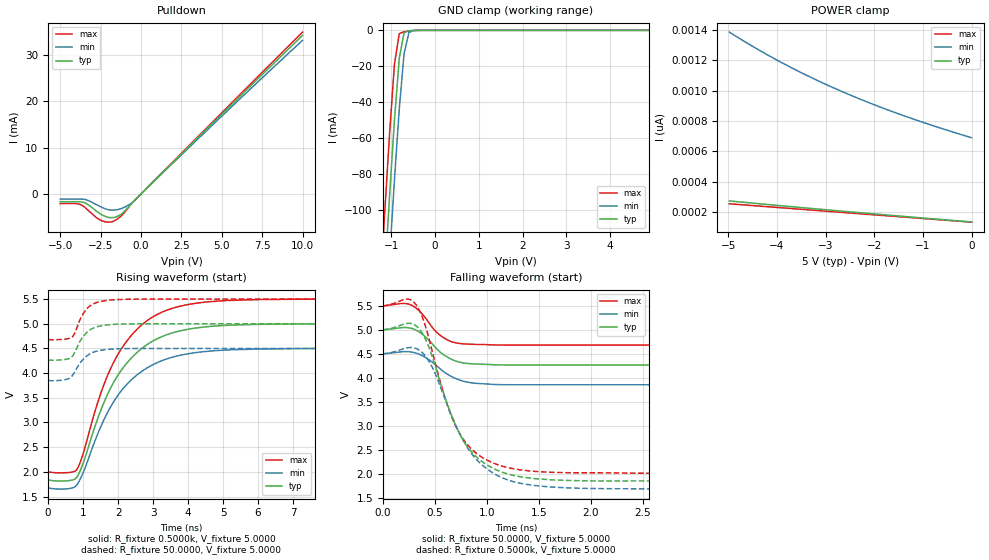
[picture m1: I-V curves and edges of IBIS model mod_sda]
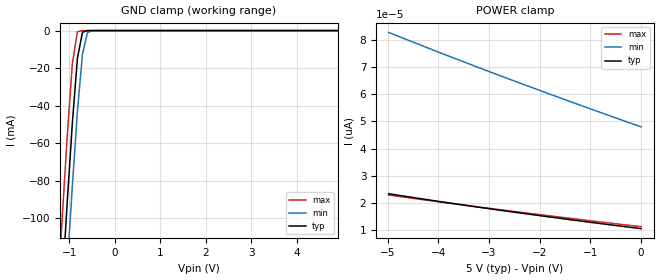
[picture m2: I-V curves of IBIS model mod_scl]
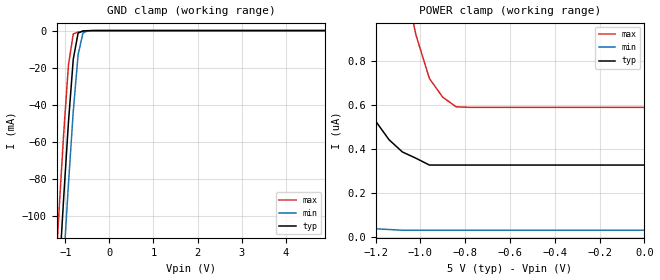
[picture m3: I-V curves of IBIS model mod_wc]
| IBIS (I/O, Buffer, Information, Specification) Model, officially
| electronic behavioral standard for Buffer structures of digital pins.
[IBIS ver]  4.0
[File name] m24c16_fc3_tssop8.ibs
[File Rev]  1.0
[Date]   24 Sept 2014
[Source]   CAD & Design Services (Catania) - STMicroelectronics
[Notes]
   (Note1)  This IBIS model includes the TSSOP8 package data
   (Note2)  This IBIS model has some Notes about the non-monotonicity
   of the I-V curves, but they are not indicative of problems
   inside the model;
[Copyright] (c) 2014 STMicroelectronics
|   Component M24C16
[Component] M24C16
[Manufacturer] STMicroelectronics
[Package]
| variable   typ   min   max
R_pkg   0.0   0.0   0.0
L_pkg   0.0H   0.0H   0.0H
C_pkg   0.0F   0.0F   0.0F
[Pin]  signal_name   model_name   R_pin   L_pin   C_pin
1   1NC   NC   NA   NA   NA
2   2NC   NC   NA   NA   NA
3   3NC   NC   NA   NA   NA
4   VSS   GND   NA   NA   NA
5   SDA   mod_sda   NA   NA   NA
6   SCL   mod_scl   NA   NA   NA
7   WCN   mod_wc   NA   NA   NA
8   VCC   POWER   NA   NA   NA
[Package Model]  182696_TSSOP8
[Define Package Model]  182696_TSSOP8
[Manufacturer]  STMicroelectronics
[OEM]  STMicroelectronics
[Description]  8 pin TSSOP package
[Number Of Pins]  8
[Pin Numbers]
|Pin Num   Terminal Name
1   | net1
2   | net2
3   | net3
4   | net4_GND
5   | net5
6   | net6
7   | net7
8   | net8_VDD
[Model Data]
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[End Model Data]
[End Package Model]
| Models and submodels in the file (3): mod_sda (I/O_open_drain), mod_scl (Input), mod_wc (Input)
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|   Model mod_sda
[Model]   mod_sda
Model_type I/O_open_drain
Polarity   Inverting
Vinl   =   1.500V
Vinh   =   3.500V
Vmeas  =   2.500V
Cref   =   10pF
Rref   =   1k
Vref   =   5.000V
C_comp   1.845pF   1.683pF   1.932pF
[Temperature Range]  25.0000   85.0000   -40.0000
[Voltage Range]   5.0000V   4.5000V   5.5000V
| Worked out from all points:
|   slope of the pulldown table from 0 to 0.75 V, typ, clamps not added: 290 ohm
|   GND clamp passes 1 mA (typ) near -0.68 V on its own axis
|   rising waveform, R_fixture 0.5000k, V_fixture 5.0000: 20-80 % time 1.33ns typ, 1.36ns min, 1.29ns max; typ from 1.83 V to 5 V
|   rising waveform, R_fixture 50.0000, V_fixture 5.0000: 20-80 % time 396ps typ, 424ps min, 373ps max; typ from 4.27 V to 5 V
|   falling waveform, R_fixture 50.0000, V_fixture 5.0000: 20-80 % time 226ps typ, 256ps min, 202ps max; typ from 5 V to 4.27 V
|   falling waveform, R_fixture 0.5000k, V_fixture 5.0000: 20-80 % time 361ps typ, 392ps min, 333ps max; typ from 5 V to 1.83 V
[Pulldown]
|Voltage   I(typ)   I(min)   I(max)
-5V       -1.67mA    -1.12mA    -2.076mA
-4.04V    -1.67mA    -1.12mA    -2.076mA
-3.72V    -1.69mA    -1.124mA   -2.322mA
-3.4V     -2.033mA   -1.24mA    -3.126mA
-2.76V    -3.71mA    -2.317mA   -5.101mA
-2.28V    -4.74mA    -3.122mA   -5.95mA
-1.8V     -5.117mA   -3.496mA   -6.006mA
-1.48V    -4.87mA    -3.399mA   -5.446mA
-1.16V    -4.184mA   -3.077mA   -4.516mA
-520mV    -1.838mA   -1.762mA   -1.845mA
5.24V     18.02mA    17.57mA    18.34mA
10V       34.18mA    33.1mA     34.88mA
[GND_clamp]
|Voltage   I(typ)   I(min)   I(max)
-5V       -1.825A    -1.857A    -1.794A
-1.26V    -181mA     -216.2mA   -145.7mA
-1.15V    -135.5mA   -170.6mA   -100.2mA
-1.04V    -91.23mA   -126mA     -56.63mA
-930mV    -49.7mA    -83.07mA   -18.72mA
-820mV    -15.43mA   -43.63mA   -1.793mA
-710mV    -1.308mA   -12.96mA   -800.3uA
-600mV    -197.9uA   -1.278mA   -438.8uA
-490mV    -52.7uA    -150.8uA   -129uA
4.9V      130.6pA    728.2pA    117.6pA
[POWER_clamp]
|Voltage   I(typ)   I(min)   I(max)
-4.98V    272.3pA    1.386nA    253.4pA
-4.44V    256pA      1.28nA     240.1pA
-3.84V    238.3pA    1.174nA    225.3pA
-3.3V     222.7pA    1.087nA    212.1pA
-2.7V     205.8pA    998.7pA    197.5pA
-2.04V    187.6pA    911.4pA    181.4pA
-1.38V    169.7pA    832.6pA    165.4pA
-660mV    150.5pA    754.6pA    148pA
0V        133.2pA    689.1pA    132pA
[Ramp]
| variable   typ   min   max
dV/dt_r   0.4405/0.4439n   0.3885/0.4693n   0.4915/0.4754n
dV/dt_f   0.4405/0.2435n   0.3885/0.2716n   0.4915/0.2233n
R_load = 50.0000
[Rising Waveform]
R_fixture= 0.5000k
V_fixture= 5.0000
V_fixture_min= 4.5000
V_fixture_max= 5.5000
|time   V(typ)   V(min)   V(max)
0s        1.835V     1.675V     1.998V
830ps     1.903V     1.747V     2.059V
1.01ns    2.192V     1.996V     2.39V
1.49ns    3.219V     2.891V     3.561V
1.89ns    3.834V     3.439V     4.244V
2.41ns    4.328V     3.885V     4.79V
3.11ns    4.694V     4.211V     5.186V
3.95ns    4.882V     4.386V     5.383V
4.98ns    4.963V     4.464V     5.465V
10ns      5V         4.5V       5.5V
[Rising Waveform]
R_fixture= 50.0000
V_fixture= 5.0000
V_fixture_min= 4.5000
V_fixture_max= 5.5000
|time   V(typ)   V(min)   V(max)
0s        4.266V     3.852V     4.681V
470ps     4.276V     3.866V     4.688V
670ps     4.324V     3.932V     4.721V
750ps     4.406V     4.012V     4.795V
950ps     4.691V     4.239V     5.141V
1.13ns    4.841V     4.362V     5.32V
1.37ns    4.933V     4.441V     5.425V
1.73ns    4.979V     4.482V     5.477V
2.75ns    4.999V     4.499V     5.499V
10ns      5V         4.5V       5.5V
[Falling Waveform]
R_fixture= 50.0000
V_fixture= 5.0000
V_fixture_min= 4.5000
V_fixture_max= 5.5000
|time   V(typ)   V(min)   V(max)
0s        5V         4.5V       5.5V
200ps     5.047V     4.543V     5.55V
280ps     5.027V     4.535V     5.511V
420ps     4.833V     4.41V      5.22V
500ps     4.647V     4.283V     4.988V
580ps     4.487V     4.135V     4.843V
680ps     4.365V     4.005V     4.738V
840ps     4.293V     3.898V     4.699V
1.26ns    4.266V     3.853V     4.681V
10ns      4.266V     3.852V     4.681V
[Falling Waveform]
R_fixture= 0.5000k
V_fixture= 5.0000
V_fixture_min= 4.5000
V_fixture_max= 5.5000
|time   V(typ)   V(min)   V(max)
0s        5V         4.5V       5.5V
230ps     5.132V     4.621V     5.641V
320ps     5.083V     4.611V     5.525V
400ps     4.852V     4.478V     5.148V
480ps     4.414V     4.2V       4.511V
620ps     3.457V     3.436V     3.434V
740ps     2.825V     2.831V     2.832V
960ps     2.242V     2.169V     2.333V
1.28ns    1.952V     1.818V     2.091V
10ns      1.835V     1.675V     1.998V
|   Model mod_scl
[Model]   mod_scl
Model_type Input
Vinl   =   1.500V
Vinh   =   3.500V
C_comp   1.762pF   1.683pF   1.932pF
[Temperature Range]  25.0000   85.0000   -40.0000
[Voltage Range]   5.0000V   4.5000V   5.5000V
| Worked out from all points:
|   GND clamp passes 1 mA (typ) near -0.71 V on its own axis
[GND_clamp]
|Voltage   I(typ)   I(min)   I(max)
-5V       -1.81A     -1.842A    -1.778A
-1.26V    -178.8mA   -214.1mA   -143mA
-1.15V    -133.6mA   -168.8mA   -97.85mA
-1.04V    -89.77mA   -124.5mA   -54.7mA
-930mV    -48.59mA   -81.99mA   -17.17mA
-820mV    -14.68mA   -42.87mA   -624.4uA
-710mV    -882.5uA   -12.5mA    -4.426uA
-600mV    -18.77uA   -1.029mA   -29.45nA
-490mV    -372.8nA   -42.06uA   -196.9pA
4.9V      10.41pA    50.62pA    10.07pA
[POWER_clamp]
|Voltage   I(typ)   I(min)   I(max)
-4.98V    23.46pA    82.67pA    22.99pA
-3.78V    20.06pA    73.87pA    19.98pA
-2.58V    16.89pA    65.38pA    17.13pA
-1.38V    13.9pA     57.16pA    14.39pA
0V        10.64pA    47.99pA    11.36pA
|   Model mod_wc
[Model]   mod_wc
Model_type Input
Vinl   =   1.500V
Vinh   =   3.500V
C_comp   1.762pF   1.683pF   1.932pF
[Temperature Range]  25.0000   85.0000   -40.0000
[Voltage Range]   5.0000V   4.5000V   5.5000V
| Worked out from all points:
|   GND clamp passes 1 mA (typ) near -0.68 V on its own axis
[GND_clamp]
|Voltage   I(typ)   I(min)   I(max)
-5V       -1.825A    -1.857A    -1.794A
-1.26V    -181mA     -216.2mA   -145.7mA
-1.15V    -135.5mA   -170.6mA   -100.2mA
-1.04V    -91.23mA   -126mA     -56.63mA
-930mV    -49.7mA    -83.07mA   -18.72mA
-820mV    -15.43mA   -43.63mA   -1.793mA
-710mV    -1.308mA   -12.96mA   -800.3uA
-600mV    -197.9uA   -1.278mA   -438.8uA
-490mV    -52.7uA    -150.8uA   -129uA
4.9V      130.6pA    728.2pA    117.6pA
[POWER_clamp]
|Voltage   I(typ)   I(min)   I(max)
-4.98V    12.45uA    7.203uA    21.47uA
-2.04V    3.072uA    934.7nA    6.194uA
-1.62V    1.738uA    210.8nA    4.139uA
-1.56V    1.528uA    130.8nA    3.799uA
-1.44V    1.128uA    70.7nA     3.191uA
-1.38V    924.7nA    50.4nA     2.845uA
-1.32V    757.7nA    41.6nA     2.511uA
-1.14V    442.5nA    33.5nA     1.521uA
-1.02V    358.3nA    30.2nA     920.4nA
-960mV    327.1nA    30.2nA     721.9nA
-840mV    327.1nA    30.2nA     592.2nA
0V        327.1nA    30.2nA     589.9nA
